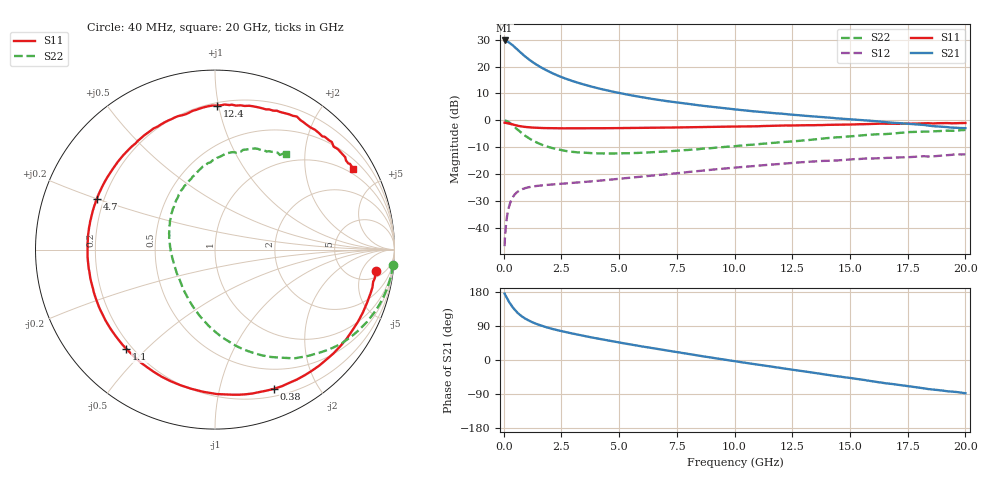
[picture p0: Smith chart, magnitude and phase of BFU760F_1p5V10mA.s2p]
! Filename:  P:\Prog\Test\Noise\ATS_data\Testdata_Net\Split files Spar\BFU760F_2W_C1_Bias3_1.5V_5mA_60mA_D.s2p
! Date/Time: Mon 06/Feb/2012 15:06:56
! BFU760_2W_C1_Bias3_1.5V_5mA_60mA_R.s2p
! MDIF S-parameter v. bias file
! BFU760_2W_C1_1.5V_5mA_60mA
! Date/time Fri Mar 18 11:09:37 2011
! VAR V_out= 1.5001
! VAR I_out= 9.9250
! VAR V_in= 0.7748
! VAR I_in= 0.0291
! Device data file deembeded for feedlines and parallel
! Original file: \Split files Spar\BFU760_2W_C1_Bias3_1.5V_5mA_60mA_R.s2p
! Feed-files: PR003V01_101208_Feed1.s2p, PR003V01_101208_Feed2.s2p
! Parallel-file: PR003V01_101208_Par.s2p
# MHz S MA R 50
!  Freq-MHz  S11-mag  S11-arg  S21-mag  S21-arg  S12-mag  S12-arg  S22-mag  S22-arg
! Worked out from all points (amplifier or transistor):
!   167 points, 40 MHz to 20 GHz, reference 50 ohm
!   highest |S21| = 29.7 dB at 40 MHz (marker M1)
!   |S21| within 3 dB of that: start of sweep to 546.7 MHz
!   unconditionally stable (mu >= 1): 5.255 GHz to 13.7 GHz
!   at 550 MHz: K = 0.13, MSG = 26.8 dB, |S12| = -26.9 dB
!   at 4.2 GHz: K = 0.88, MSG = 17.0 dB, |S12| = -22.4 dB
!   at 20 GHz: K = 0.85, MSG = 4.9 dB, |S12| = -12.6 dB
!   S11 on the Smith chart (normalised r, x): 40 MHz: 7, -9; 380 MHz: 0.28, -1.47; 1.1 GHz: 0.18, -0.43; 4.7 GHz: 0.17, +0.20; 12.4 GHz: 0.22, +0.99; 20 GHz: 0.80, +3.53
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40  0.904 -7.8  30.55 175.3  0.004583 85.6  0.9945 -5.1
50  0.9044 -10.2  30.53 173.6  0.006183 87.0  0.9924 -6.5
120  0.8953 -23.1  29.81 165.7  0.01361 78.3  0.9756 -15.5
220  0.8775 -41.3  28.27 154.8  0.02378 69.0  0.9259 -27.7
280  0.8642 -51.5  27.08 148.9  0.02909 64.0  0.8898 -34.3
380  0.8421 -67.2  25.07 140.1  0.03635 56.5  0.8182 -44.6
460  0.8237 -78.3  23.42 133.8  0.04104 51.5  0.765 -51.7
550  0.805 -89.2  21.57 127.7  0.04501 46.6  0.7026 -59.0
700  0.7799 -104.3  18.75 119.3  0.05009 40.4  0.6187 -69.1
900  0.7567 -120.0  15.78 110.5  0.05443 34.6  0.5293 -80.0
1100  0.7417 -131.9  13.49 103.7  0.05728 30.6  0.4632 -89.0
1450  0.7265 -147.2  10.65 94.6  0.06047 26.2  0.3841 -102.0
1900  0.7157 -160.6  8.316 85.5  0.06326 23.3  0.3239 -115.2
2500  0.7111 -173.3  6.375 76.2  0.06626 21.7  0.2806 -129.8
3400  0.7113 172.7  4.736 64.5  0.07118 20.6  0.2519 -146.5
4700  0.7165 156.8  3.436 49.5  0.07962 20.3  0.2424 -166.9
6800  0.7312 135.9  2.369 27.7  0.0971 17.8  0.2609 167.2
10200  0.7699 106.8  1.569 -5.0  0.134 6.8  0.338 132.1
12400  0.8018 89.1  1.289 -24.7  0.1604 -3.8  0.4032 112.1
13400  0.8108 81.7  1.183 -33.4  0.1719 -10.2  0.4392 103.7
16800  0.8642 55.2  0.9055 -63.1  0.2016 -30.8  0.5653 75.2
20000  0.8923 30.3  0.7156 -87.8  0.2331 -52.4  0.6626 53.5
